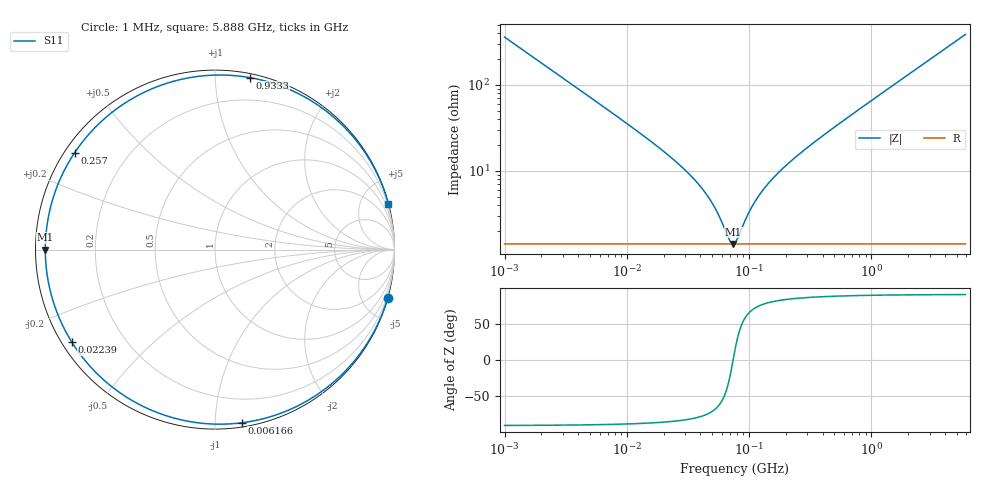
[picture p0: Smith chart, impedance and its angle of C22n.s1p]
!Extracted from simulation file : D:\simuICEMC\chap5\exo_decap_mounting\Capa_22n.spc
# HZ Z MA R 50
!freq magS11 phS11
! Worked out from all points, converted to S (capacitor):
!   378 points, 1 MHz to 5.888 GHz, reference 50 ohm
!   read as one part to ground: C = 440 pF near 1.023 MHz
!   lowest |Z| = 1.4 ohm at 74.13 MHz (marker M1)
!   series resonance near 74.05 MHz, so ESL is about 10 nH
!   S11 on the Smith chart (normalised r, x): 1 MHz: 0.03, -7.23; 6.166 MHz: 0.03, -1.17; 22.39 MHz: 0.03, -0.29; 257 MHz: 0.03, +0.31; 933.3 MHz: 0.03, +1.22; 5.888 GHz: 0.03, +7.77
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1000000  7.233 -89.8
1862087  3.883 -89.6
2398833  3.013 -89.5
3019952  2.392 -89.3
4265795  1.69 -89.1
6165950  1.165 -88.6
7413102  0.9665 -88.3
8912509  0.8004 -88.0
1.122018e7  0.6306 -87.5
1.412538e7  0.4943 -86.8
1.778279e7  0.3844 -85.8
2.238721e7  0.2949 -84.6
2.630268e7  0.242 -83.4
4.168694e7  0.1218 -76.7
7.413102e7  0.028 0.4
7.762471e7  0.02948 18.2
1.412538e8  0.138 78.3
2.290868e8  0.2721 84.1
2.570396e8  0.3123 84.9
3.311311e8  0.416 86.1
4.168694e8  0.5334 87.0
5.370318e8  0.6957 87.7
6.76083e8  0.8818 88.2
9.332543e8  1.224 88.7
1.380384e9  1.816 89.1
1.995262e9  2.629 89.4
3.162278e9  4.17 89.6
5.888437e9  7.768 89.8
